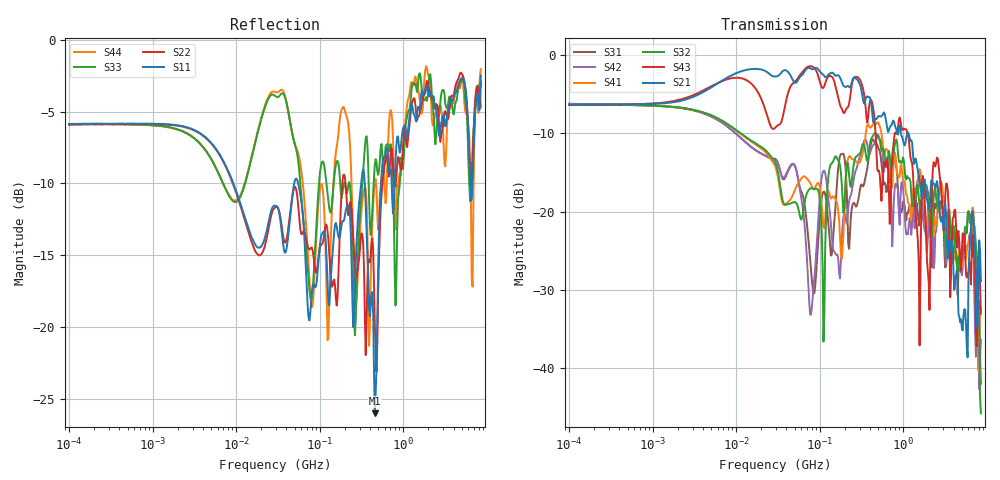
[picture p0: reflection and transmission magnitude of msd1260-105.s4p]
# MHz S MA R 50
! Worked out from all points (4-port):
!   498 points, 100 kHz to 8.5 GHz, reference 50 ohm
!   strongest paths, dB at 100 kHz, 1.698 MHz, 29.49 MHz, 500.7 MHz, 8.5 GHz:
!     S21: -6.3, -6.0, -2.7, -7.8, -28.9
!     S43: -6.3, -5.9, -9.2, -14.8, -33.0
!     S32: -6.4, -6.6, -13.8, -10.6, -45.8
!     S41: -6.4, -6.6, -14.3, -8.6, -32.4
!     S42: -6.2, -6.6, -13.4, -10.2, -36.4
!     S31: -6.2, -6.6, -13.3, -11.8, -42.0
!   lowest |S11| = -26.0 dB at 457 MHz (marker M1), VSWR 1.11, Z = 54.9 - j1.95 ohm
!   |S11| at or under -10 dB: 55.24 MHz to 313.6 MHz (258.4 MHz wide, 140 % of centre); 346.2 MHz to 543.1 MHz (196.9 MHz wide, 44.3 % of centre); 6.332 GHz to 6.728 GHz (396.3 MHz wide, 6.07 % of centre)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
0.1  0.5089 4.1  0.4825 5.5  0.4883 -5.8  0.4812 -176.2
     0.4825 5.5  0.5075 4.1  0.481 -176.2  0.4907 -5.9
     0.4883 -5.8  0.481 -176.2  0.5075 4.3  0.4828 5.3
     0.4812 -176.2  0.4907 -5.9  0.4828 5.3  0.506 4.3
78.73314  0.1212 -9.1  0.8196 -15.2  0.04249 -91.2  0.1487 59.6
          0.8196 -15.2  0.189 -19.6  0.1414 74.5  0.02198 -171.4
          0.04249 -91.2  0.1414 74.5  0.1244 -18.7  0.8504 -13.8
          0.1487 59.6  0.02198 -171.4  0.8504 -13.8  0.1221 -36.3
456.9518  0.05007 -20.7  0.3883 -82.4  0.2743 -32.3  0.3638 -35.2
          0.3883 -82.4  0.1011 -44.3  0.3166 -31.7  0.2729 -30.8
          0.2743 -32.3  0.3166 -31.7  0.367 -23.5  0.3703 -128.8
          0.3638 -35.2  0.2729 -30.8  0.3703 -128.8  0.3241 -17.2
1970.81  0.6811 -165.0  0.1125 113.4  0.1325 141.1  0.1013 175.5
         0.1125 113.4  0.7143 -165.3  0.1236 135.5  0.06806 179.6
         0.1325 141.1  0.1236 135.5  0.642 -157.9  0.04144 143.9
         0.1013 175.5  0.06806 179.6  0.04144 143.9  0.7603 -174.1
3651.237  0.6147 15.0  0.05895 -171.8  0.08178 -9.8  0.06388 -17.3
          0.05895 -171.8  0.6106 5.6  0.08209 -10.4  0.08463 -20.4
          0.08178 -9.8  0.08209 -10.4  0.6149 -3.8  0.02843 145.0
          0.06388 -17.3  0.08463 -20.4  0.02843 145.0  0.5792 -3.3
6920.76  0.3969 47.7  0.08974 -18.4  0.06395 13.5  0.09938 49.8
         0.08974 -18.4  0.468 24.8  0.08252 41.9  0.05569 -6.0
         0.06395 13.5  0.08252 41.9  0.4814 18.6  0.05178 -3.1
         0.09938 49.8  0.05569 -6.0  0.05178 -3.1  0.2782 56.8
8500  0.751 -32.7  0.03593 -140.9  0.007958 -105.8  0.02402 -56.7
      0.03593 -140.9  0.7137 -42.1  0.005147 -66.3  0.01521 -55.9
      0.007958 -105.8  0.005147 -66.3  0.5813 -48.7  0.02232 -122.6
      0.02402 -56.7  0.01521 -55.9  0.02232 -122.6  0.7895 -39.7
